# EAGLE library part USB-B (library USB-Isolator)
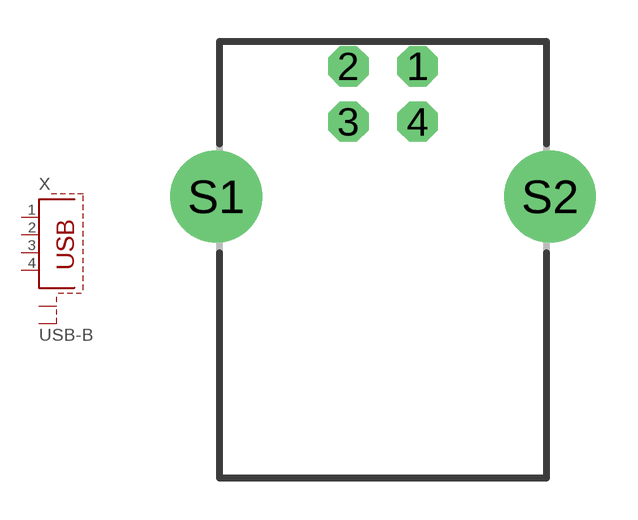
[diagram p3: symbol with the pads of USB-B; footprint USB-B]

Designator prefix X

## USB-B (OC_FARNELL: unknown; OC_NEWARK: unknown)  [USB-B]
1  1  pas
2  2  pas
3  3  pas
4  4  pas
S1  S1  pas
S2  S2  pas

## Footprint USB-B (pad centres in mm)
USB connector with shield
drill 0.95 octagon: 1 1.25,4.71; 2 -1.25,4.71; 3 -1.25,2.71; 4 1.25,2.71
drill 2.3 pad 2.9: S1 -6.02,0; S2 6.02,0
